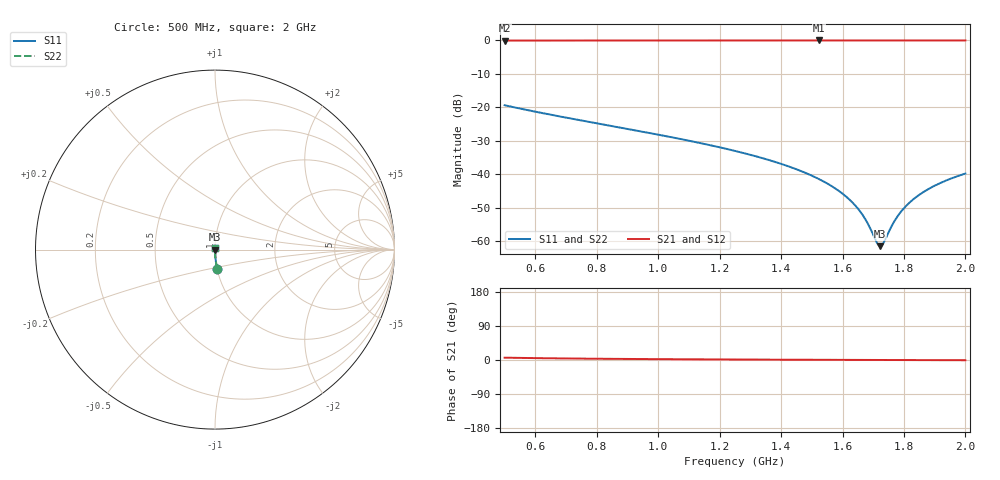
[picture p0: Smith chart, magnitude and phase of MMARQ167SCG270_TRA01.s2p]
! MMARQ167SCG270_TRA01  S-PARAMETER MODEL  ( General Type )
! Model Generated by TAIYO YUDEN Corporation (http://www.ty-top.com)
! Version 1.0
! TAIYO YUDEN Control No. 160201
! Copyright(c) 2016 TAIYO YUDEN CO.,LTD. All Rights Reserved.
! Product Description (link to TY-COMPAS)
! https://ds.yuden.co.jp/TYCOMPAS/or/detail?pn=MMARQ167SCG270JTRA01&u=M
! Products Name : Multilayer Ceramic Capacitors
! Characteristics :
!  Capacitance : 27 pF , Rated Voltage : 250V , TCC : CG / C0G
!  Case Size : 1.6 x 0.8 / 0.063 x 0.031 [mm/inch] , Thickness : 0.7 / 0.028 [mm/inch]
!  (Conditions: Temperature = 25 degC , DC Bias Current/Voltage = 0A / 0V)
! External Node Assignments :
!  1  o---| |---o  2
! GND o---------o GND
! Frequency Range : 500MHz  -  2000MHz  [ 401 STEP ]
# MHz S RI R 50
! Freq[MHz].  S11 Real  S11 Imag  S21 Real  S21 Imag  S12 Real  S12 Imag  S22 Real  S22 Imag
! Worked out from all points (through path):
!   401 points, 500 MHz to 2 GHz, reference 50 ohm
!   highest |S21| = -0.01 dB at 1.524 GHz (marker M1); lowest = -0.1 dB at 500 MHz (marker M2)
!   group delay of S21, straight-line fit = 10.9 ps
!   lowest |S11| = -61.5 dB at 1.722 GHz (marker M3), VSWR 1.00, Z = 50.1 - j0.00233 ohm
!   |S11| at or under -10 dB: start of sweep to end of sweep
!   |S22| runs from -61.5 to -19.4 dB; largest |S21 - S12| = 0
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500  0.0119 -0.1067  0.9881 0.1067  0.9881 0.1067  0.0119 -0.1067
751.25  0.00448 -0.0632  0.9955 0.0632  0.9955 0.0632  0.00448 -0.0632
1002.5  0.00207 -0.0387  0.9979 0.0387  0.9979 0.0387  0.00207 -0.0387
1250  0.00115 -0.0222  0.9988 0.0222  0.9988 0.0222  0.00115 -0.0222
1392.5  0.000927 -0.0146  0.9991 0.0146  0.9991 0.0146  0.000927 -0.0146
1501.25  0.000843 -0.00941  0.9992 0.00941  0.9992 0.00941  0.000843 -0.00941
1523.75  0.000833 -0.00839  0.9992 0.00839  0.9992 0.00839  0.000833 -0.00839
1587.5  0.000818 -0.00558  0.9992 0.00558  0.9992 0.00558  0.000818 -0.00558
1636.25  0.000818 -0.00352  0.9992 0.00352  0.9992 0.00352  0.000818 -0.00352
1670  0.000822 -0.00213  0.9992 0.00213  0.9992 0.00213  0.000822 -0.00213
1685  0.000826 -0.00152  0.9992 0.00152  0.9992 0.00152  0.000826 -0.00152
1711.25  0.000833 -0.000469  0.9992 0.000469  0.9992 0.000469  0.000833 -0.000469
1722.5  0.000837 -2.33e-05  0.9992 2.33e-05  0.9992 2.33e-05  0.000837 -2.33e-05
1733.75  0.000842 0.000419  0.9992 -0.000419  0.9992 -0.000419  0.000842 0.000419
1752.5  0.00085 0.00115  0.9992 -0.00115  0.9992 -0.00115  0.00085 0.00115
1771.25  0.000859 0.00187  0.9991 -0.00187  0.9991 -0.00187  0.000859 0.00187
1790  0.000869 0.00259  0.9991 -0.00259  0.9991 -0.00259  0.000869 0.00259
1812.5  0.000883 0.00344  0.9991 -0.00344  0.9991 -0.00344  0.000883 0.00344
1842.5  0.000903 0.00456  0.9991 -0.00456  0.9991 -0.00456  0.000903 0.00456
1876.25  0.000928 0.00579  0.9991 -0.00579  0.9991 -0.00579  0.000928 0.00579
1913.75  0.000959 0.00714  0.999 -0.00714  0.999 -0.00714  0.000959 0.00714
2000  0.00104 0.0102  0.999 -0.0102  0.999 -0.0102  0.00104 0.0102
